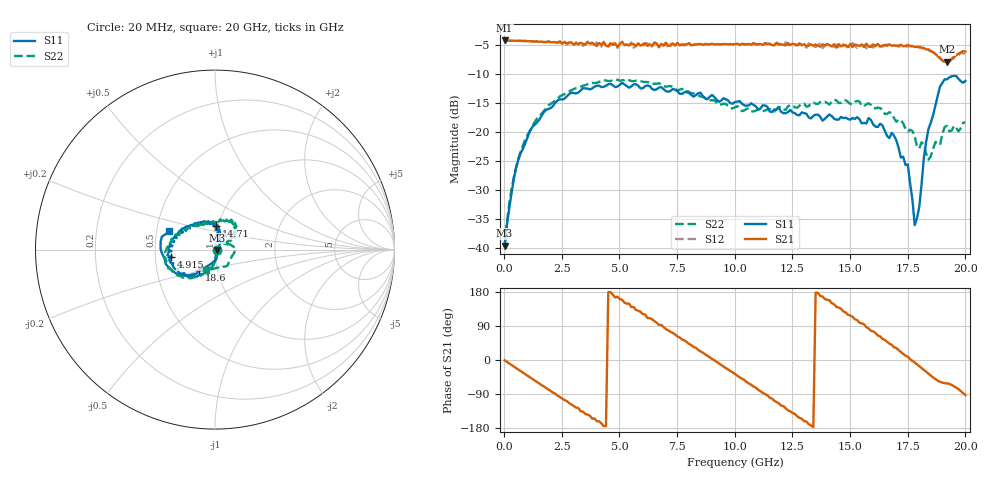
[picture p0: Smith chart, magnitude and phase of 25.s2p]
!Agilent Technologies,N5230A,US43500223,A.07.50.48
!Agilent N5230A: A.07.50.48
!Date: Monday, September 14, 2015 12:02:09
!Correction: S11(Full 2 Port(1,2))
!S21(Full 2 Port(1,2))
!S12(Full 2 Port(1,2))
!S22(Full 2 Port(1,2))
!S2P File: Measurements: S11, S21, S12, S22:
# Hz S  dB  R 50
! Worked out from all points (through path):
!   201 points, 20 MHz to 20 GHz, reference 50 ohm
!   highest |S21| = -4.17 dB at 20 MHz (marker M1); lowest = -7.8 dB at 19.2 GHz (marker M2)
!   group delay of S21, straight-line fit = 113 ps
!   lowest |S11| = -39.6 dB at 20 MHz (marker M3), VSWR 1.02, Z = 51 - j0.194 ohm
!   |S11| at or under -10 dB: start of sweep to end of sweep
!   |S22| runs from -39.7 to -10.9 dB; largest |S21 - S12| = 0.066
!   S11 on the Smith chart (normalised r, x): 20 MHz: 1.02, -0.00; 4.915 GHz: 0.61, -0.05; 14.71 GHz: 0.98, +0.26; 18.6 GHz: 0.82, -0.19; 20 GHz: 0.58, +0.13
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2e7  -39.58 -10.4  -4.17 -0.8  -4.18 -0.8  -39.69 -3.8
4.196e8  -28.11 -73.3  -4.22 -17.3  -4.23 -17.3  -27.78 -76.5
9.191e8  -21.86 -95.5  -4.25 -37.5  -4.26 -37.7  -21.24 -96.2
2.1179e9  -15.48 -122.0  -4.46 -86.1  -4.34 -85.4  -14.87 -122.6
3.4166e9  -12.40 -146.5  -4.74 -136.2  -5.11 -137.3  -11.98 -145.0
4.3157e9  -12.18 -162.3  -4.49 -174.3  -4.41 -170.8  -11.01 -158.2
4.9151e9  -12.12 -170.3  -5.31 167.1  -5.46 165.5  -10.96 -165.6
6.7133e9  -12.30 168.0  -5.35 92.6  -5.28 92.5  -11.54 172.5
8.4116e9  -13.30 151.2  -4.85 26.9  -4.77 25.5  -13.67 149.0
1.001e10  -14.81 132.0  -4.81 -37.1  -4.80 -38.0  -15.68 118.8
1.18082e10  -16.09 105.9  -4.58 -111.0  -4.61 -111.2  -16.03 86.5
1.34066e10  -17.18 92.8  -5.07 -176.8  -5.11 179.8  -14.90 68.3
1.47053e10  -17.57 87.0  -4.98 128.3  -4.82 129.6  -14.51 56.0
1.57043e10  -18.51 87.4  -4.74 87.0  -5.51 88.0  -15.18 46.6
1.67033e10  -21.02 81.1  -4.84 43.1  -5.18 42.1  -16.55 38.5
1.75025e10  -25.60 53.2  -4.95 8.7  -5.26 6.1  -19.93 26.4
1.78022e10  -36.05 -5.1  -5.31 -6.6  -5.35 -7.9  -20.70 33.8
1.8002e10  -32.84 -65.0  -5.28 -16.2  -5.40 -17.8  -22.79 23.5
1.83017e10  -21.58 -106.0  -5.71 -30.9  -5.55 -33.2  -23.73 37.9
1.86014e10  -17.02 -128.0  -6.18 -46.2  -6.20 -47.7  -22.83 28.0
1.92008e10  -10.89 -169.5  -7.82 -61.7  -8.06 -64.8  -18.92 -4.2
2e10  -11.15 157.8  -6.08 -92.6  -6.39 -94.6  -18.27 -112.9
